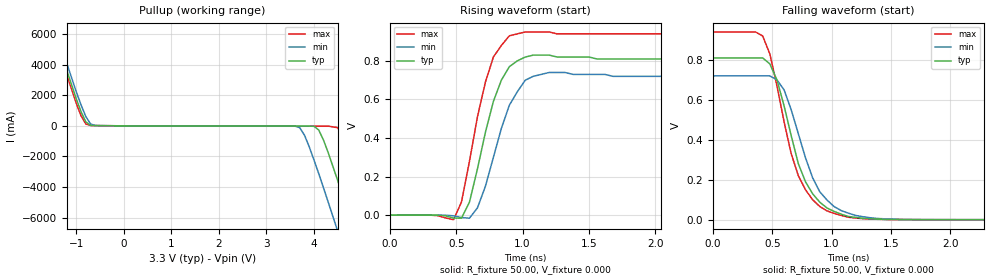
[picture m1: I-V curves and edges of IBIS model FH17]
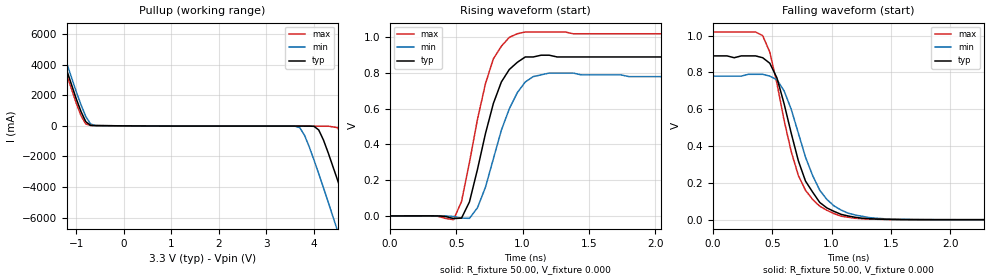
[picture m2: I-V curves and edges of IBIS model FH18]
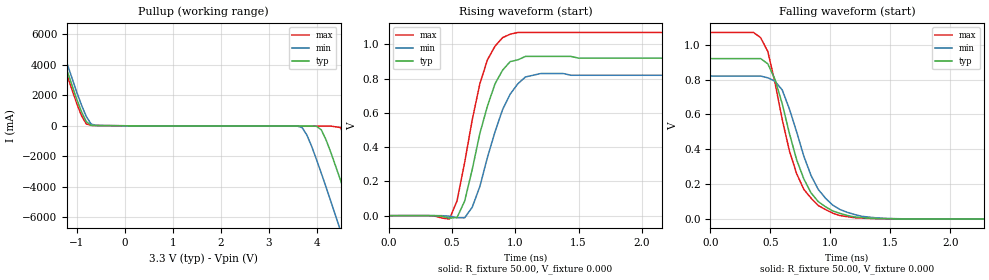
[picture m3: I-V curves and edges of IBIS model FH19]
|   * 932sq420d.ibs * IBIS 3.2 Model file
| Rev History
| Rev No.   Description
| 1.0   Initial release with Updated Parasitic Parameters
| 1.1   Updated Vmeas parameters
| 1.2   Replaced ICS with IDT in disclaimer, updated copyright
[IBIS Ver]   3.2
[Comment char]  |_char
[File name]   932sq420d.ibs
[Date]   Sept 27, 2010
[File Rev]   1.1
[Source]   Originated at Integrated Device Technology, Inc.
[Disclaimer] (C) Copyright Integrated Device Technology, Inc. 2010
   All rights reserved
IDT hereby grants the user of this IBIS model a non-exclusive,
nontransferable license to use this IBIS model under the following terms.
Before using this IBIS model, the user should read this license.
If the user does not accept these terms,  the IBIS model should be
returned to IDT within 30 days.
   The user is granted this license only to use the IBIS model and
is not granted rights to sell, load, rent, lease or license the IBIS
model in whole or in part, or in modified form to anyone other than
user. User may modify the IBIS model to suit its specific
applications but rights to derivative works and such modifications
shall belong to IDT.
   This IBIS model is provided on an "AS IS" basis and IDT makes
absolutely no warranty with respect to the information contained
herein. IDT DISCLAIMS AND CUSTOMER WAIVES ALL WARRANTIES, EXPRESS
OR IMPLIED, INCLUDING WARRANTIES OF MERCHANTABILITY OR FITNESS FOR
A PARTICULAR PURPOSE. The entire risk as to quality and performance
is with the Customer. ACCORDINGLY, IN NO EVENT SHALL THE COMPANY BE
LIABLE FOR ANY DAMAGES, WHETHER IN CONTRACT OR TORT,INCLUDING ANY
LOST PROFITS OR OTHER INCIDENTAL, CONSEQUENTIAL, EXEMPLARY, OR
PUNITIVE DAMAGES ARISING OUT OF THE USE OR APPLICATION OF THE IBIS
model provided in this package. Further, IDT reserves the right to
make changes without notice to any product herein to improve
reliability, function, or design. IDT does not convey any license
under patent rights or any other intellectual property rights,
including those of third parties.
   IDT is not obligated to provide maintenance or support
for the licensed IBIS model.
|   COMPONENT: ICS932SQ420DG
[Component]   ICS932SQ420DG
[Manufacturer]  IDT
[Package]   |TSSOP
| variable   typ   min   max
R_pkg   81.1m   62.2m   100.0m
L_pkg   6.7nH   4.9nH   8.5nH
C_pkg   0.53pF  0.21pF  0.85pF
[Pin]   signal_name   model_name   R_pin   L_pin   C_pin
  1   SMBCLK   FI4
  2   AGND14   GND
  3   AVDD14   POWER
  4   VDD14   POWER
  5   **REF14_3x/TEST_SEL   FIO49
  6   GND14   GND
  7   GNDXTAL   GND
  8   X1_25   FIX
  9   X2_25   FIX
 10   VDDXTAL   POWER
 11   GNDPCI   GND
 12   VDDPCI   POWER
 13   PCI4_2x   FO2X
 14   PCI3_2x   FO2X
 15   PCI2_2x   FO2X
 16   PCI1_2x   FO2X
 17   PCI0_2x   FO2X
 18   GNDPCI   GND
 19   VDDPCI   POWER
 20   VDD48   POWER
 21   *48M_2x/100M_133M#   FIO48
 22   GND48   GND
 23   AGND96   GND
 24   DOT96T   CK410
 25   DOT96C   CK410
 26   AVDD96   POWER
 27   TEST_MODE   FI3
 28   CKPWRGD#/PD   FI1
 29   VDDSRC   POWER
 30   SRC0T   CK410
 31   SRC0C   CK410
 32   GNDSRC   GND
 33   SRC1C   CK410
 34   SRC1T   CK410
 35   SRC2C   CK410
 36   SRC2T   CK410
 37   VDDSRC   POWER
 38   AVDD_SRC   POWER
 39   AGND_SRC   GND
 40   IREF   NC
 41   NS_SRC0C   CK410
 42   NS_SRC0T   CK410
 43   NS_SRC1C   CK410
 44   NS_SRC1T   CK410
 45   VDDNS   POWER
 46   GNDNS   GND
 47   NS_SAS0C   CK410
 48   NS_SAS0T   CK410
 49   NS_SAS1C   CK410
 50   NS_SAS1T   CK410
 51   AVDD_NS_SAS   POWER
 52   AGNDNS   GND
 53   CPU0C   CK410
 54   CPU0T   CK410
 55   CPU1C   CK410
 56   CPU1T   CK410
 57   VDDCPU   POWER
 58   GNDCPU   GND
 59   CPU2C   CK410
 60   CPU2T   CK410
 61   CPU3C   CK410
 62   CPU3T   CK410
 63   VDDCPU   POWER
 64   SMBDAT   FIOD1
|* Either 3.3V or 2.5V
|** All model are simulated with typical corner process
[Diff Pin]   inv_pin   vdiff   tdelay_typ
24   25   NA   NA
30   31   NA   NA
34   33   NA   NA
36   35   NA   NA
42   41   NA   NA
44   43   NA   NA
48   47   NA   NA
50   49   NA   NA
54   53   NA   NA
56   55   NA   NA
60   59   NA   NA
62   61   NA   NA
[Model Selector] CK410
FH17   100ohm differential output trace. 475ohm on IREF pin.
FH18   85ohm differential output trace. 432ohm on IREF pin.
FH19   85ohm differential output trace. 412ohm on IREF pin.
| Models and submodels in the file (11): FH17 (Open_source), FH18 (Open_source), FH19 (Open_source), FI1 (Input), FI3 (Input), FI4 (Input), FIX (Input), FIOD1 (I/O_open_drain), FO2X (Output), FIO48 (I/O), FIO49 (I/O)
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|   Model FH17
[Model]   FH17
Model_type   Open_source
Polarity   Inverting
Vmeas =   1.50V
Rref =  0.000
Vref =   1.50V
C_comp   3.40pF   2.85pF   3.95pF
[Temperature Range]   27.00   70.00   0.000
[Voltage Range]   3.30V   3.00V   3.70V
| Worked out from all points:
|   slope of the pullup table from 0 to 0.495 V, typ, clamps not added: 52.3 ohm
|   rising waveform, R_fixture 50.00, V_fixture 0.000: 20-80 % time 179ps typ, 188ps min, 175ps max; typ from 0 V to 0.81 V
|   falling waveform, R_fixture 50.00, V_fixture 0.000: 20-80 % time 244ps typ, 252ps min, 238ps max; typ from 0.81 V to 0 V
[Pullup]
| voltage   I(typ)   I(min)   I(max)
-3.3V     24.08A     24.51A     23.82A
-1.7V     8.35A      8.81A      8.07A
-1.5V     6.42A      6.89A      6.13A
-900mV    930mA      1.37A      660mA
-700mV    30.96mA    120mA      21.99mA
3.7V      -16.39mA   -120mA     -18.9mA
4.1V      -270mA     -3.12A     -18.94mA
4.5V      -3.58A     -6.89A     -120mA
4.7V      -5.47A     -8.82A     -1.48A
4.9V      -7.4A      -10.76A    -3.29A
5.3V      -11.29A    -14.67A    -7.11A
6.6V      -24.11A    -27.5A     -19.88A
[Ramp]
| variable   typ   min   max
dV/dt_r   0.49/0.18n   0.43/0.19n   0.56/0.17n
dV/dt_f   0.49/0.24n   0.43/0.26n   0.56/0.23n
R_load = 50.00
[Rising Waveform]
R_fixture = 50.00
V_fixture = 0.000
V_fixture_min = 0.000
V_fixture_max = 0.000
| time   V(typ)   V(min)   V(max)
0s        -30.52uV   -28.4uV    -32.6uV
480ps     -15mV      -3.17mV    -23.17mV
540ps     -15.18mV   -12.27mV   68.75mV
600ps     67.96mV    -15.34mV   280mV
660ps     240mV      38.04mV    510mV
780ps     590mV      300mV      820mV
900ps     770mV      570mV      930mV
1.02ns    820mV      700mV      950mV
1.2ns     830mV      740mV      950mV
3ns       810mV      720mV      940mV
[Falling Waveform]
R_fixture = 50.00
V_fixture = 0.000
V_fixture_min = 0.000
V_fixture_max = 0.000
| time   V(typ)   V(min)   V(max)
0s        810mV      720mV      940mV
420ps     810mV      720mV      920mV
480ps     780mV      720mV      830mV
600ps     570mV      650mV      490mV
720ps     280mV      430mV      220mV
840ps     130mV      210mV      99.86mV
960ps     59.06mV    99.23mV    44.35mV
1.08ns    27.64mV    45.82mV    21.42mV
1.38ns    3.04mV     6.23mV     2.13mV
3ns       -12.4uV    12.33uV    6.65uV
|   Model FH18
[Model]   FH18
Model_type   Open_source
Polarity   Inverting
Vmeas =   1.50V
Rref =  0.000
Vref =   1.50V
C_comp   3.40pF   2.85pF   3.95pF
[Temperature Range]   27.00   70.00   0.000
[Voltage Range]   3.30V   3.00V   3.70V
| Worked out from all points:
|   slope of the pullup table from 0 to 0.495 V, typ, clamps not added: 50.5 ohm
|   rising waveform, R_fixture 50.00, V_fixture 0.000: 20-80 % time 188ps typ, 198ps min, 179ps max; typ from 0 V to 0.89 V
|   falling waveform, R_fixture 50.00, V_fixture 0.000: 20-80 % time 247ps typ, 259ps min, 234ps max; typ from 0.89 V to 0 V
[Pullup]
| voltage   I(typ)   I(min)   I(max)
-3.3V     24.08A     24.52A     23.82A
-1.7V     8.36A      8.82A      8.07A
-1.5V     6.42A      6.89A      6.14A
-900mV    930mA      1.37A      660mA
-700mV    31.27mA    120mA      22.29mA
3.7V      -17.85mA   -120mA     -20.6mA
4.1V      -270mA     -3.13A     -20.64mA
4.5V      -3.58A     -6.9A      -120mA
4.7V      -5.48A     -8.83A     -1.48A
4.9V      -7.4A      -10.77A    -3.29A
5.3V      -11.29A    -14.68A    -7.12A
6.6V      -24.11A    -27.51A    -19.89A
[Ramp]
| variable   typ   min   max
dV/dt_r   0.53/0.18n   0.47/0.20n   0.61/0.17n
dV/dt_f   0.53/0.24n   0.47/0.26n   0.61/0.23n
R_load = 50.00
[Rising Waveform]
R_fixture = 50.00
V_fixture = 0.000
V_fixture_min = 0.000
V_fixture_max = 0.000
| time   V(typ)   V(min)   V(max)
0s        -30.53uV   -28.41uV   -32.61uV
480ps     -14.93mV   -3.16mV    -21.09mV
540ps     -12.41mV   -12.19mV   80.59mV
600ps     78.84mV    -13.71mV   300mV
660ps     260mV      45.46mV    540mV
780ps     630mV      320mV      880mV
900ps     820mV      600mV      1V
1.02ns    890mV      750mV      1.03V
1.2ns     900mV      800mV      1.03V
3ns       890mV      780mV      1.02V
[Falling Waveform]
R_fixture = 50.00
V_fixture = 0.000
V_fixture_min = 0.000
V_fixture_max = 0.000
| time   V(typ)   V(min)   V(max)
0s        890mV      780mV      1.02V
420ps     880mV      790mV      1V
480ps     850mV      780mV      910mV
540ps     770mV      760mV      740mV
600ps     630mV      700mV      540mV
720ps     320mV      470mV      240mV
840ps     150mV      240mV      110mV
960ps     63.84mV    110mV      51.1mV
1.38ns    3.22mV     7.52mV     2.32mV
3ns       4.51uV     12.3uV     10.28uV
|   Model FH19
[Model]   FH19
Model_type   Open_source
Polarity   Inverting
Vmeas =   1.50V
Rref =  0.000
Vref =   1.50V
C_comp   3.40pF   2.85pF   3.95pF
[Temperature Range]   27.00   70.00   0.000
[Voltage Range]   3.30V   3.00V   3.70V
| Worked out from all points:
|   slope of the pullup table from 0 to 0.495 V, typ, clamps not added: 49.7 ohm
|   rising waveform, R_fixture 50.00, V_fixture 0.000: 20-80 % time 192ps typ, 207ps min, 183ps max; typ from 0 V to 0.92 V
|   falling waveform, R_fixture 50.00, V_fixture 0.000: 20-80 % time 247ps typ, 261ps min, 236ps max; typ from 0.92 V to 0 V
[Pullup]
| voltage   I(typ)   I(min)   I(max)
-3.3V     24.08A     24.52A     23.82A
-1.7V     8.36A      8.82A      8.07A
-1.5V     6.42A      6.89A      6.14A
-900mV    930mA      1.37A      670mA
-700mV    31.43mA    120mA      22.44mA
3.7V      -18.62mA   -120mA     -21.5mA
4.1V      -270mA     -3.13A     -21.54mA
4.5V      -3.58A     -6.9A      -120mA
4.7V      -5.48A     -8.83A     -1.48A
4.9V      -7.4A      -10.77A    -3.3A
5.3V      -11.29A    -14.68A    -7.12A
6.6V      -24.11A    -27.51A    -19.89A
[Ramp]
| variable   typ   min   max
dV/dt_r   0.55/0.19n   0.49/0.20n   0.64/0.18n
dV/dt_f   0.55/0.24n   0.49/0.26n   0.64/0.23n
R_load = 50.00
[Rising Waveform]
R_fixture = 50.00
V_fixture = 0.000
V_fixture_min = 0.000
V_fixture_max = 0.000
| time   V(typ)   V(min)   V(max)
0s        -30.53uV   -28.41uV   -32.61uV
480ps     -14.89mV   -3.15mV    -19.92mV
540ps     -10.88mV   -12.14mV   86.84mV
600ps     84.67mV    -12.81mV   310mV
660ps     270mV      49.33mV    560mV
780ps     640mV      340mV      910mV
900ps     850mV      620mV      1.04V
1.02ns    910mV      770mV      1.07V
1.2ns     930mV      830mV      1.07V
3ns       920mV      820mV      1.07V
[Falling Waveform]
R_fixture = 50.00
V_fixture = 0.000
V_fixture_min = 0.000
V_fixture_max = 0.000
| time   V(typ)   V(min)   V(max)
0s        920mV      820mV      1.07V
420ps     920mV      820mV      1.04V
480ps     890mV      810mV      960mV
540ps     800mV      790mV      780mV
600ps     660mV      740mV      570mV
720ps     340mV      500mV      260mV
840ps     150mV      250mV      120mV
960ps     70.7mV     120mV      54.46mV
1.38ns    3.55mV     7.17mV     1.98mV
3ns       -15.26uV   2.47uV     6.71uV
